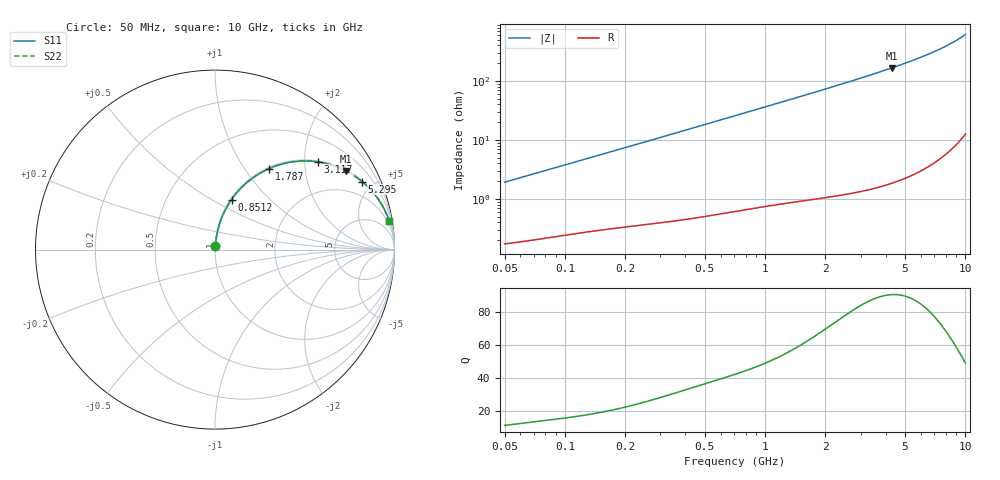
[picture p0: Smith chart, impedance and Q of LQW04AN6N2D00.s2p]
!Murata Part Number: LQW04AN6N2D00
!These Parameters are Measured in Series Mode Connection
!  o--[Z]--o
!Port1  Port2
!  o-------o
!Freq. Start=50[MHz] Stop=10[GHz], 401[Steps]
# Hz S RI R 50
!Freq.(Hz)	S 11(Real)	S 11(Imag)	S 21(Real)	S 21(Imag)	S 12(Real)	S 12(Imag)	S 22(Real)	S 22(Imag)
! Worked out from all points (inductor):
!   401 points, 50 MHz to 10 GHz, reference 50 ohm
!   read as one part in series: L = 6.05 nH near 51.34 MHz
!   highest Q = 90.6 at 4.284 GHz (marker M1), where L = 6.17 nH
!   S11 on the Smith chart (normalised r, x): 50 MHz: 1.00, +0.04; 851.2 MHz: 1.01, +0.62; 1.787 GHz: 1.02, +1.30; 3.117 GHz: 1.03, +2.33; 5.295 GHz: 1.05, +4.29; 10 GHz: 1, +12
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5e7  0.00208 0.019  0.9979 -0.019  0.9979 -0.019  0.00208 0.019
1.214486e8  0.00469 0.0451  0.9953 -0.0451  0.9953 -0.0451  0.00469 0.0451
1.956524e8  0.00842 0.0714  0.9916 -0.0714  0.9916 -0.0714  0.00842 0.0714
2.949953e8  0.0153 0.1061  0.9847 -0.1061  0.9847 -0.1061  0.0153 0.1061
4.628099e8  0.0321 0.1626  0.9679 -0.1626  0.9679 -0.1626  0.0321 0.1626
7.071068e8  0.0669 0.2383  0.9331 -0.2383  0.9331 -0.2383  0.0669 0.2383
8.511793e8  0.0922 0.2786  0.9078 -0.2786  0.9078 -0.2786  0.0922 0.2786
1.024606e9  0.1263 0.3223  0.8737 -0.3223  0.8737 -0.3223  0.1263 0.3223
1.21714e9  0.1677 0.3644  0.8323 -0.3644  0.8323 -0.3644  0.1677 0.3644
1.445853e9  0.22 0.4058  0.78 -0.4058  0.78 -0.4058  0.22 0.4058
1.717543e9  0.284 0.4432  0.716 -0.4432  0.716 -0.4432  0.284 0.4432
1.787167e9  0.3004 0.4509  0.6996 -0.4509  0.6996 -0.4509  0.3004 0.4509
2.391784e9  0.4367 0.4895  0.5633 -0.4895  0.5633 -0.4895  0.4367 0.4895
3.117263e9  0.5747 0.4886  0.4253 -0.4886  0.4253 -0.4886  0.5747 0.4886
3.606216e9  0.6495 0.4715  0.3505 -0.4715  0.3505 -0.4715  0.6495 0.4715
4.171863e9  0.7198 0.4436  0.2802 -0.4436  0.2802 -0.4436  0.7198 0.4436
4.283859e9  0.7319 0.4375  0.2681 -0.4375  0.2681 -0.4375  0.7319 0.4375
5.295127e9  0.819 0.3794  0.181 -0.3794  0.181 -0.3794  0.819 0.3794
6.374006e9  0.8801 0.3188  0.1199 -0.3188  0.1199 -0.3188  0.8801 0.3188
7.472112e9  0.921 0.2629  0.079 -0.2629  0.079 -0.2629  0.921 0.2629
8.530394e9  0.9476 0.2151  0.0524 -0.2151  0.0524 -0.2151  0.9476 0.2151
1e10  0.9712 0.1574  0.0288 -0.1574  0.0288 -0.1574  0.9712 0.1574
